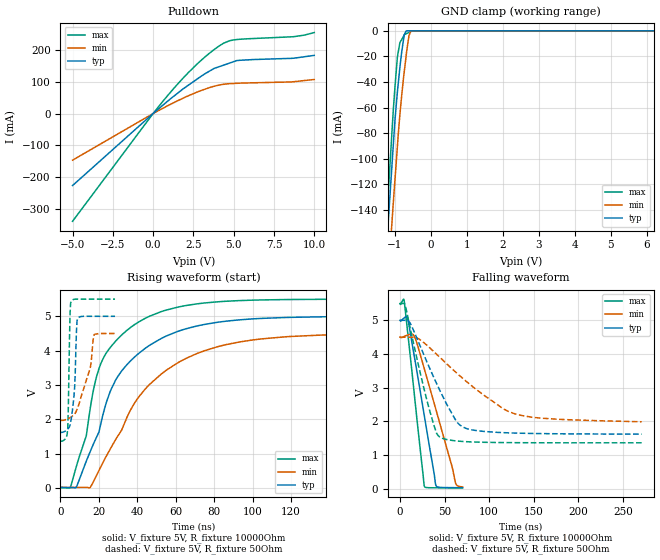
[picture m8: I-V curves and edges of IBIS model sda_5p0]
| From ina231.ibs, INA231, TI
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|   sda_5p0 Model
[Model]   sda_5p0
Model_type   I/O_open_drain
Polarity   Non-Inverting
Vinl = 0.4
Vinh = 1.4
Vmeas = 2.5
Vref = 5.0
Cref = 2pF
Rref = 10000
|   typ   min   max
|   (nom PVT)   (fast PVT)   (slow PVT)
|C_comp from frequency sweep method (F=100KHz)
|C_comp   2.313e-10   1.861e-10   4.284e-10
|ON state : BUFFER OUTPUT TURNED LOW
|C_comp   2.313e-10   1.861e-10   4.284e-10
|OFF state: BUFFER IN HIGH IMPEDANCE
|C_comp   2.199e-12   1.849e-12   2.612e-12
|C_comp from LC tank measurement(L=1nH)
|Resonant Frequency(Hz)   5.880e+09   5.890e+09   5.670e+09
C_comp   7.334e-13   7.309e-13   7.887e-13
|ON state : BUFFER OUTPUT TURNED LOW
|Resonant Frequency(Hz)   5.880e+09   5.890e+09   5.670e+09
|C_comp   7.334e-13   7.309e-13   7.887e-13
|OFF state: BUFFER IN HIGH IMPEDANCE
|Resonant Frequency(Hz)   5.100e+09   5.820e+09   4.670e+09
|C_comp   9.748e-13   7.486e-13   1.163e-12
| Where nom  PVT is Nominal Process, 5V, 27C
|   Fast PVT is Strong Process,  5.5V, -40C
|   Slow PVT is Weak Process,   4.5V, 125C
[Voltage Range]   5   4.5   5.5
|Ambient Temperature   25   150   -65
|Junction Temperature
[Temperature Range]   27   125   -40
[Pullup Reference]   5   4.5   5.5
[Pulldown Reference]   0   0   0
[Power Clamp Reference]   5   4.5   5.5
[GND Clamp Reference]   0   0   0
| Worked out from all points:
|   slope of the pulldown table from 0 to 0.75 V, typ, clamps not added: 23.1 ohm
|   GND clamp passes 1 mA (typ) near -0.71 V on its own axis
|   falling waveform, V_fixture 5V, R_fixture 10000Ohm: 20-80 % time 19ns typ, 28.5ns min, 13.3ns max; typ from 5 V to 0.024 V
|   rising waveform, V_fixture 5V, R_fixture 10000Ohm: 20-80 % time 27.5ns typ, 36.1ns min, 19.9ns max; typ from 0.011 V to 5 V
|   falling waveform, V_fixture 5V, R_fixture 50Ohm: 20-80 % time 35.6ns typ, 68.7ns min, 22.4ns max; typ from 5 V to 1.62 V
|   rising waveform, V_fixture 5V, R_fixture 50Ohm: 20-80 % time 1.89ns typ, 6.69ns min, 799ps max; typ from 1.62 V to 5 V
[Pulldown]
|   Voltage   I(typ)   I(min)   I(max)
-5V       -226.4mA   -146.6mA   -338.7mA
0V        0A         0A         0A
676mV     29.2mA     18.39mA    42.63mA
2.178V    88.69mA    55.59mA    128.1mA
2.909V    114.6mA    70.95mA    163.9mA
3.679V    138.6mA    84.21mA    196.8mA
4.378V    152.1mA    91.92mA    221.2mA
4.966V    162.5mA    94.39mA    231mA
5.395V    167.4mA    95.5mA     233.4mA
8.7V      173.8mA    99.88mA    241.4mA
9.371V    178.3mA    103.6mA    246.3mA
10V       182.7mA    107mA      254.4mA
[GND Clamp]
|   Voltage   I(typ)   I(min)   I(max)
-5V       -1.882A    -1.835A    -1.964A
-1.247V   -174.1mA   -215mA     -153.9mA
-1.051V   -90.38mA   -135.7mA   -63.1mA
-1V       -69.11mA   -115.7mA   -43.24mA
-935.5mV  -48.12mA   -90.94mA   -20.93mA
-864mV    -28.35mA   -65.46mA   -9.073mA
-815mV    -16.72mA   -50.71mA   -6.844mA
-745mV    -3.172mA   -32.34mA   -3.367mA
-690mV    -47.56uA   -19.34mA   -2.311mA
-612.5mV  0A         -3.853mA   -1.239mA
-558.5mV  0A         -6.961uA   -491.3uA
10V       0A         0A         0A
[POWER Clamp]
|   Voltage   I(typ)   I(min)   I(max)
-5V       0A         0A         0A
0V        0A         0A         0A
10V       0A         0A         0A
[Ramp]
R_load = 10000
|   typ   min   max
dV/dt_r   2.99325/2.7454e-08   2.69033/3.60483e-08   3.29489/1.99143e-08
dV/dt_f   2.98709/1.8962e-08   2.68429/2.86549e-08   3.28889/1.3288e-08
[Falling Waveform]
V_fixture = 5V
V_fixture_min = 4.5V
V_fixture_max = 5.5V
R_fixture = 10000Ohm
|   Time   V(typ)   V(min)   V(max)
0s        5V         4.5V       5.5V
4.1ns     5.058V     4.515V     5.632V
5ns       5.079V     4.526V     5.537V
8.6ns     5.061V     4.565V     4.66V
15.8ns    3.977V     4.544V     2.884V
27.2ns    2.186V     3.571V     78.58mV
40.4ns    84.06mV    2.341V     20.95mV
58.4ns    25.58mV    649.3mV    19.54mV
62.3ns    24.86mV    163.4mV    19.41mV
70.2ns    23.76mV    44.89mV    19.16mV
[Rising Waveform]
V_fixture = 5V
V_fixture_min = 4.5V
V_fixture_max = 5.5V
R_fixture = 10000Ohm
|   Time   V(typ)   V(min)   V(max)
0s        11.24mV    16.04mV    8.51mV
5.3ns     6.209mV    12.73mV    29.08mV
13.4ns    770.4mV    15.69mV    1.506V
15.5ns    1.058V     13.79mV    2.317V
23.3ns    2.378V     864.3mV    3.882V
32.9ns    3.479V     1.826V     4.509V
53ns      4.369V     3.341V     5.146V
81.8ns    4.826V     4.114V     5.423V
117.2ns   4.966V     4.403V     5.488V
299.9ns   5V         4.5V       5.5V
[Falling Waveform]
V_fixture = 5V
V_fixture_min = 4.5V
V_fixture_max = 5.5V
R_fixture = 50Ohm
|   Time   V(typ)   V(min)   V(max)
0s        5V         4.5V       5.5V
5.9ns     5.003V     4.502V     5.447V
11.9ns    4.896V     4.501V     4.721V
32.3ns    3.639V     4.21V      2.416V
41ns      3.127V     3.994V     1.648V
45.8ns    2.857V     3.873V     1.511V
62.3ns    2.041V     3.465V     1.417V
70.1ns    1.837V     3.282V     1.399V
128.3ns   1.649V     2.226V     1.363V
270.9ns   1.617V     1.985V     1.359V
[Rising Waveform]
V_fixture = 5V
V_fixture_min = 4.5V
V_fixture_max = 5.5V
R_fixture = 50Ohm
|   Time   V(typ)   V(min)   V(max)
0s        1.617V     1.967V     1.36V
3.8ns     1.712V     2.013V     1.741V
5ns       1.827V     2.046V     5.09V
5.6ns     2.001V     2.067V     5.436V
7.4ns     2.937V     2.15V      5.498V
8.3ns     4.525V     2.242V     5.5V
8.9ns     4.933V     2.323V     5.501V
15.5ns    5V         3.496V     5.5V
17.6ns    5V         4.469V     5.5V
28.4ns    5V         4.5V       5.5V
